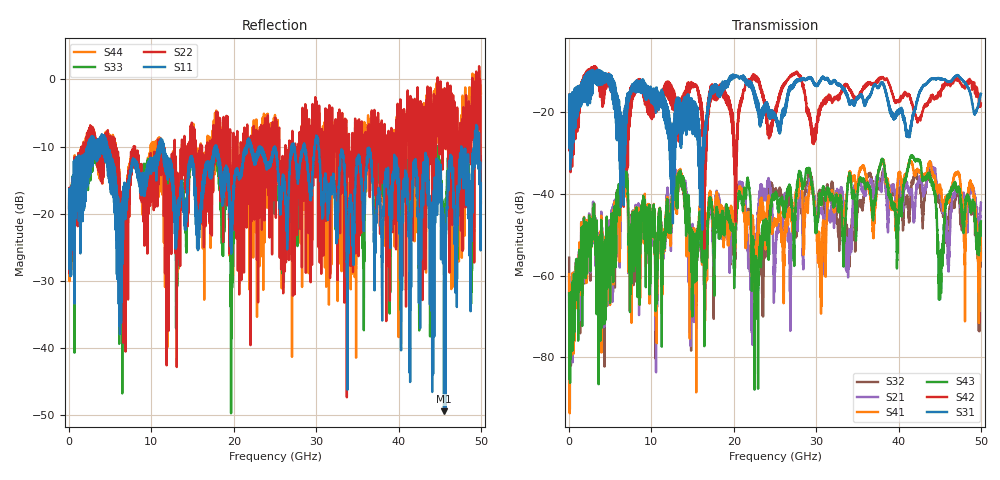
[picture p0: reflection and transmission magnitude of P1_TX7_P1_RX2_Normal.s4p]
!Keysight Technologies,N5225B,MY57041031,A.13.20.10
!Date: Friday, May 31, 2019 11:16:03
!Correction: S11(Full 4 Port(1,2,3,4))
!S12(Full 4 Port(1,2,3,4))
!S13(Full 4 Port(1,2,3,4))
!S14(Full 4 Port(1,2,3,4))
!S21(Full 4 Port(1,2,3,4))
!S22(Full 4 Port(1,2,3,4))
!S23(Full 4 Port(1,2,3,4))
!S24(Full 4 Port(1,2,3,4))
!S31(Full 4 Port(1,2,3,4))
!S32(Full 4 Port(1,2,3,4))
!S33(Full 4 Port(1,2,3,4))
!S34(Full 4 Port(1,2,3,4))
!S41(Full 4 Port(1,2,3,4))
!S42(Full 4 Port(1,2,3,4))
!S43(Full 4 Port(1,2,3,4))
!S44(Full 4 Port(1,2,3,4))
!S4P File: Measurements: <S11,S12,S13,S14>,
!<S21,S22,S23,S24>,
!<S31,S32,S33,S34>,
!<S41,S42,S43,S44>:
# Hz S  dB  R 50.0
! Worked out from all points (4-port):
!   5000 points, 10 MHz to 50 GHz, reference 50 ohm
!   strongest paths, dB at 10 MHz, 12.51 GHz, 25.01 GHz, 37.51 GHz, 50 GHz:
!     S31: -19.4, -39.2, -20.9, -14.0, -15.5
!     S42: -19.4, -16.3, -19.7, -12.6, -17.9
!     S43: -64.3, -42.7, -41.1, -35.3, -46.8
!     S41: -59.7, -43.2, -46.5, -35.3, -53.3
!     S21: -60.6, -41.5, -59.2, -36.6, -42.1
!     S32: -55.6, -41.3, -39.3, -37.9, -54.0
!   lowest |S11| = -49.4 dB at 45.52 GHz (marker M1), VSWR 1.01, Z = 49.8 + j0.233 ohm
!   |S11| at or under -10 dB: 4.613 GHz to 10.86 GHz (6.246 GHz wide, 80.7 % of centre); 11.46 GHz to 17.74 GHz (6.279 GHz wide, 43 % of centre); 30.28 GHz to 47.62 GHz (17.33 GHz wide, 44.5 % of centre)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
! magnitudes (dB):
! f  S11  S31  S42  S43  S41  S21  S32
! 10 MHz  -19.1  -19.4  -19.4  -64.3  -59.7  -60.6  -55.6
! 6.47 GHz  -22.2  -23.3  -27.3  -32.2  -33.7  -34.2  -32.5
! 21.75 GHz  -9.3  -12.9  -12.3  -37.0  -45.5  -58.2  -44.4
! 22.75 GHz  -11.5  -18.5  -11.9  -57.3  -52.0  -54.6  -58.3
! 28.99 GHz  -12.8  -11.9  -19.7  -34.5  -44.7  -40.9  -37.0
! 45.52 GHz  -49.4  -11.9  -13.2  -49.0  -42.3  -42.9  -45.2
! 50 GHz  -15.5  -15.5  -17.9  -46.8  -53.3  -42.1  -54.0
